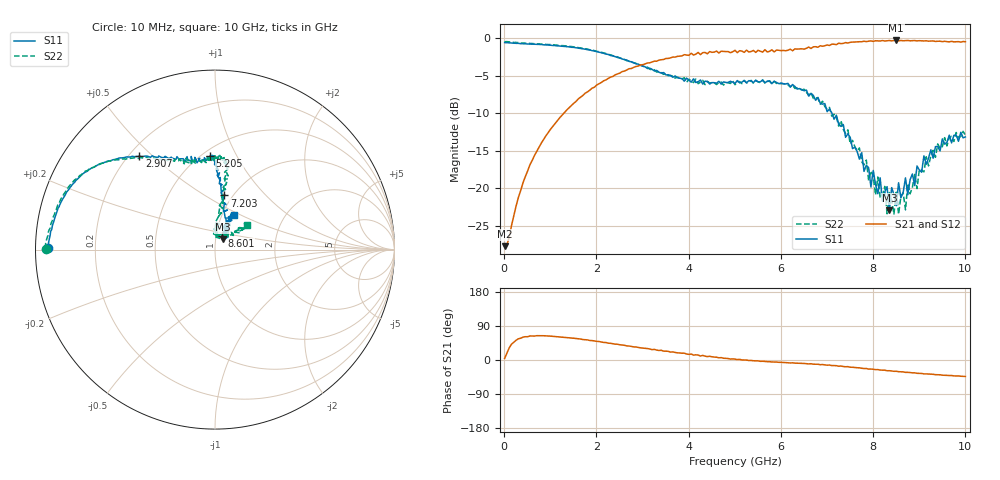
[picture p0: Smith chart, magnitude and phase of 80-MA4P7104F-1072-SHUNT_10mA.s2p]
!Agilent Technologies,E8364C,MY48140145,A.09.42.15
!Agilent E8364C: A.09.42.15
!Date: Wednesday, December 02, 2020 11:06:42
!Correction: S11(Full 2 Port(1,2))
!S21(Full 2 Port(1,2))
!S12(Full 2 Port(1,2))
!S22(Full 2 Port(1,2))
!S2P File: Measurements: S11, S21, S12, S22:
# Hz S  dB  R 50
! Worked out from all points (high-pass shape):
!   201 points, 10 MHz to 10 GHz, reference 50 ohm
!   highest |S21| = -0.33 dB at 8.502 GHz (marker M1); lowest = -27.7 dB at 10 MHz (marker M2)
!   |S21| within 3 dB of the highest: 3.105 GHz to end of sweep
!   lowest |S11| = -22.9 dB at 8.352 GHz (marker M3), VSWR 1.15, Z = 54.1 + j6.24 ohm
!   |S11| at or under -10 dB: 7.107 GHz to end of sweep
!   |S22| runs from -23.4 to -0.5 dB; largest |S21 - S12| = 0.031
!   S11 on the Smith chart (normalised r, x): 10 MHz: 0.03, +0.01; 2.907 GHz: 0.24, +0.45; 5.205 GHz: 0.55, +0.79; 7.203 GHz: 0.92, +0.61; 8.601 GHz: 1.06, +0.17; 10 GHz: 1.13, +0.46
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1e7  -0.61 179.3  -27.68 4.2  -27.03 -5.9  -0.50 179.6
6.5935e8  -0.84 167.9  -15.60 63.2  -15.59 63.9  -0.76 167.6
1.7083e9  -1.42 150.3  -7.64 53.9  -7.58 54.3  -1.38 150.7
2.9071e9  -3.48 129.0  -3.73 33.2  -3.69 33.2  -3.56 130.1
3.35665e9  -4.56 120.0  -2.94 25.2  -3.03 25.8  -4.44 122.0
5.005e9  -6.05 91.9  -1.64 2.3  -1.57 1.6  -6.22 92.8
5.2048e9  -5.65 92.9  -1.91 -0.1  -1.94 0.3  -5.64 91.1
6.7033e9  -7.64 88.3  -1.18 -11.1  -1.14 -10.3  -8.04 82.5
7.2028e9  -10.27 80.2  -0.88 -15.0  -0.84 -15.5  -10.49 82.9
7.95205e9  -19.82 59.9  -0.39 -23.9  -0.44 -24.3  -17.69 82.2
8.05195e9  -19.46 66.0  -0.37 -25.5  -0.39 -24.7  -20.87 83.0
8.25175e9  -20.48 43.2  -0.40 -26.9  -0.37 -27.5  -19.74 89.0
8.3017e9  -19.77 57.7  -0.38 -28.3  -0.32 -27.5  -23.37 84.9
8.35165e9  -22.89 53.1  -0.34 -28.2  -0.37 -28.8  -20.54 73.9
8.45155e9  -20.83 62.4  -0.34 -29.8  -0.34 -29.3  -23.40 67.1
8.5015e9  -22.29 46.9  -0.33 -29.7  -0.37 -30.5  -20.32 73.8
8.55145e9  -19.25 51.8  -0.38 -30.9  -0.31 -30.4  -23.43 77.4
8.6014e9  -21.25 64.3  -0.33 -31.3  -0.37 -31.1  -21.09 56.9
8.7013e9  -18.60 59.1  -0.36 -32.6  -0.31 -31.8  -22.86 55.6
8.75125e9  -20.85 62.5  -0.33 -32.6  -0.38 -32.9  -19.37 54.0
9.1009e9  -15.67 62.6  -0.39 -36.6  -0.36 -35.6  -17.81 37.8
1e10  -13.16 61.6  -0.50 -43.4  -0.49 -43.5  -12.94 38.1
